{attribute 'call_after_init'}
FUNCTION_BLOCK FB_DS_IED_LD1_LLN0_DS4 EXTENDS FB_AcsiCommonDataSetClass
VAR
END_VAR

METHOD OnInit : BOOL
VAR
END_VAR
IF NOT DeleteAllMembers() THEN RETURN; END_IF
IF NOT AddMember(ipData:=fbIED.IEDLD1.LEDGGIO1.AnOut1, eFc:=E_AcsiFc.MX) THEN RETURN; END_IF
IF NOT AddMember(ipData:=fbIED.IEDLD1.LEDGGIO2.AnOut1, eFc:=E_AcsiFc.MX) THEN RETURN; END_IF
IF NOT AddMember(ipData:=fbIED.IEDLD1.LEDGGIO3.AnOut1, eFc:=E_AcsiFc.MX) THEN RETURN; END_IF
IF NOT AddMember(ipData:=fbIED.IEDLD1.LEDGGIO4.AnOut1, eFc:=E_AcsiFc.MX) THEN RETURN; END_IF
IF NOT AddMember(ipData:=fbIED.IEDLD1.LEDGGIO5.AnOut1, eFc:=E_AcsiFc.MX) THEN RETURN; END_IF
IF NOT AddMember(ipData:=fbIED.IEDLD1.LEDGGIO6.AnOut1, eFc:=E_AcsiFc.MX) THEN RETURN; END_IF
IF NOT AddMember(ipData:=fbIED.IEDLD1.LEDGGIO7.AnOut1, eFc:=E_AcsiFc.MX) THEN RETURN; END_IF
IF NOT AddMember(ipData:=fbIED.IEDLD1.LEDGGIO8.AnOut1, eFc:=E_AcsiFc.MX) THEN RETURN; END_IF
OnInit:= TRUE;
END_METHOD

END_FUNCTION_BLOCK
